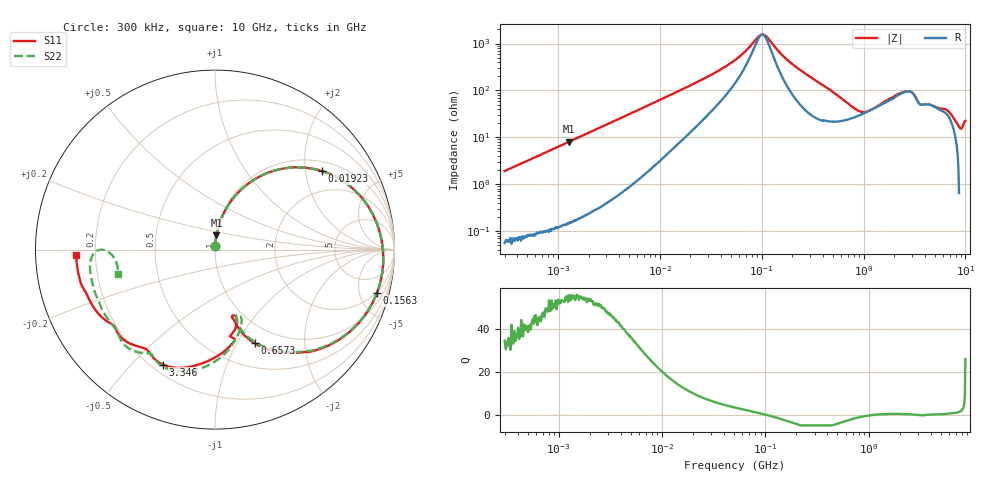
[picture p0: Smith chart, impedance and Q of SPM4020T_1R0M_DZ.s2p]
! S-Parameter Data Generated by TDK Corporation
! Copyright(C) 2024 TDK Corporation.
! All Rights Reserved.
! TDK P/N: SPM4020T-1R0M-DZ (SMD / SMT Inductor (Coil))
! Property: L=1uH at 100kHz
! Size(LxWxT): 4.3x4.1x2mm
! Model Type: s2p (Touchstone File Format Version 1.0)
! Frequency: DC=Yes Start=0.3MHz Stop=10000MHz 802points Log-sweep
! Model Generated on May 28, 2024
! Terms and conditions regarding TDK Simulation Models:
! 1)This simulation model is being provided solely for informational
!  purposes. Please refer to the specifications of the products in
!  terms of detailed characteristics of such products.
! 2)In no event shall TDK Corporation of any of its subsidiaries be
!  liable for any loss or damage arising, directly or indirectly,
!  from any information contained in this simulation model, including,
!  but not limited to loss or damages arising from any inaccuracies,
!  omissions or errors in connection with such information.
! 3)Any and all copyrights on this simulation model are owned by
!  TDK Corporation.  Duplication or redistribution of this simulation
!  model without prior written permission from TDK Corporation
!  is prohibited.
! 4)This simulation model is subject to any modification or change
!  without any prior notice.
! 5)Neither TDK Corporation nor any of its subsidiaries shall make any
!  warranty, express or implied, including but not limited to the
!  correctness, implied warranties of merchantability and fitness for
!  a particular purpose with respect to this simulation models.
! 6)The use of this simulation model shall be deemed to have consented
!  to the terms and conditions hereof.
! Port Assignments:
!  1 ---@@@--- 2
! Applicable Conditions:
!  Temperature = 25 degC
!  DC Bias Current = 0 A
!  Small Signal Operation
# Hz S MA R 50
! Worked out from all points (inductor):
!   801 points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, 300 kHz to 10 GHz, reference 50 ohm
!   read as one part in series: L = 1.01 uH near 318.3 kHz
!   highest Q = 55.1 at 1.288 MHz (marker M1), where L = 994 nH
!   self-resonance near 101.2 MHz
!   S11 on the Smith chart (normalised r, x): 300 kHz: 1.00, +0.04; 19.23 MHz: 1.28, +2.47; 156.3 MHz: 1.89, -7.13; 657.3 MHz: 0.77, -1.19; 3.346 GHz: 0.24, -0.62; 10 GHz: 0.13, -0.02
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300000  0.01952 87.7  0.9992 -1.1  0.9988 -1.1  0.01954 88.5
1288123  0.07981 84.3  0.9953 -4.6  0.9953 -4.6  0.07979 84.4
1713600  0.1057 82.8  0.9924 -6.1  0.9924 -6.1  0.1057 82.9
4734969  0.2794 72.0  0.9525 -16.4  0.9527 -16.4  0.2794 72.1
9671944  0.5051 56.5  0.8388 -30.7  0.8391 -30.7  0.505 56.5
1.922666e7  0.7397 36.2  0.6052 -48.2  0.6054 -48.2  0.7396 36.3
5.477226e7  0.9139 9.0  0.2069 -62.2  0.207 -62.2  0.9139 9.1
1.014901e8  0.9399 -4.3  0.06012 -3.3  0.06014 -3.3  0.9399 -4.2
1.563148e8  0.934 -15.0  0.1564 54.6  0.1564 54.6  0.934 -14.7
3.126428e8  0.8411 -38.2  0.4283 43.5  0.4284 43.5  0.8409 -37.7
4.568044e8  0.7191 -53.2  0.574 26.8  0.5741 26.8  0.7182 -52.7
6.573376e8  0.5678 -66.9  0.6716 6.8  0.6717 6.8  0.5645 -66.4
9.903836e8  0.427 -74.3  0.6838 -18.3  0.6839 -18.3  0.4148 -73.1
1.339606e9  0.3851 -75.8  0.6128 -36.7  0.6129 -36.7  0.3877 -69.7
1.767019e9  0.4432 -74.5  0.5298 -53.7  0.53 -53.7  0.4697 -72.9
2.446702e9  0.5882 -87.8  0.3732 -68.7  0.3733 -68.7  0.6118 -88.4
3.34571e9  0.7029 -114.3  0.3241 -64.2  0.3242 -64.2  0.7096 -115.8
3.874538e9  0.6748 -124.7  0.343 -79.0  0.343 -79.1  0.6847 -122.4
6.41458e9  0.7175 -145.6  0.2605 -117.8  0.2606 -117.8  0.7088 -142.8
8.211115e9  0.7579 -161.6  0.1877 -147.4  0.1877 -147.5  0.7068 -167.5
9.217363e9  0.7726 -169.6  0.1432 -161.1  0.1435 -161.0  0.658 -179.4
1e10  0.7765 -177.9  0.1158 -158.4  0.1157 -158.5  0.5575 -165.6
